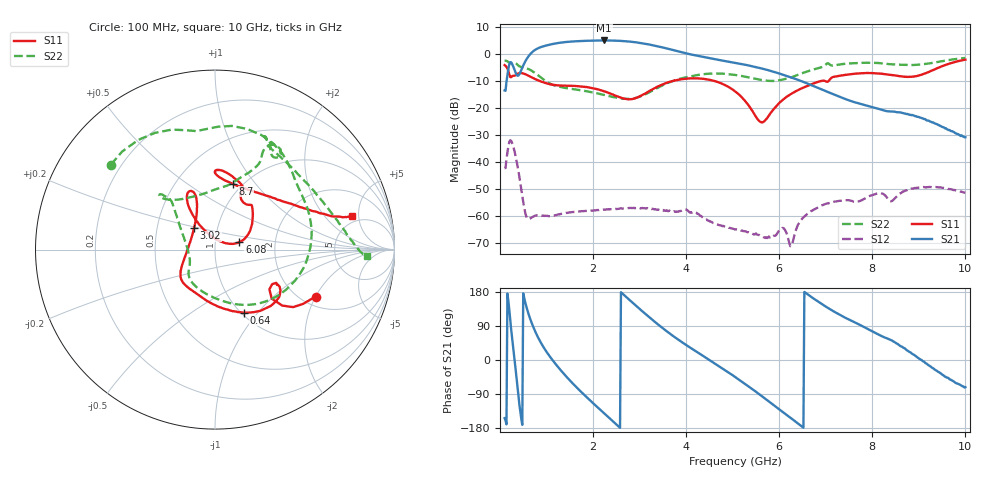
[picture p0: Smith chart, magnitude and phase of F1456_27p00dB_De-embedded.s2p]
! Integrated Device Technology
! Corporate Headquarters
! 6024 Silver Creek Valley Road
! San Jose, CA 95138  USA
! Phone:  1-408-284-8200
! Toll Free:  1-800-223-1366
! Webpage:  http://www.idt.com/
! Timing and RF Division
! 515 Groton Road, Suite 102
! Westford, MA 01886-6024
! Device:  F1456
! Description: 6-bit 0.5 dB Transmit Variable Gain Amplifier
! Frequency:  2100.0 -  2950.00 MHz
! Package:  6x6 mm Thin QFN Plastic Package: 28 pin
! State:  54
! Atten State:  27.0 dB
! Voltage:  +5.00 Volts
! Current:  216.965 mA
! Data:  The device was measured on a the F1455 evaluation board which has
!  individual transmission lines to the RF pins.  Data was collected
!  using a calibrated network analyzer.  The evaluation board was
!  de-embedded using a TRL calibration technique.
!  The reference plane is the edge of the package pin.
!  Pin  1 = CSb
!  Pin  2 = DATA
!  Pin  3 = CLK
!  Pin  4 = RSET
!  Pin  5 = GND
!  Pin  6 = RFIN  = Port 1
!  Pin  7 = GND
!  Pin  8 = NC
!  Pin  9 = NC
!  Pin 10 = NC
!  Pin 11 = NC
!  Pin 12 = NC
!  Pin 13 = NC
!  Pin 14 = /STBY
!  Pin 15 = GND
!  Pin 16 = RFOUT  = Port 2
!  Pin 17 = GND
!  Pin 18 = NC
!  Pin 19 = NC
!  Pin 20 = NC
!  Pin 21 = GND
!  Pin 22 = NC
!  Pin 23 = GND
!  Pin 24 = NC
!  Pin 25 = NC
!  Pin 26 = NC
!  Pin 27 = GND
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# GHz S dB R 50
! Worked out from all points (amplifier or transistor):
!   496 points, 100 MHz to 10 GHz, reference 50 ohm
!   highest |S21| = 5.0 dB at 2.24 GHz (marker M1)
!   |S21| within 3 dB of that: 805.4 MHz to 3.593 GHz (2.787 GHz wide, 127 % of centre)
!   unconditionally stable (mu >= 1): start of sweep to end of sweep
!   at 1.74 GHz: K = 210.59, MAG = 5.3 dB, |S12| = -58.3 dB
!   at 5.06 GHz: K = 1041.17, MAG = -2.3 dB, |S12| = -65.1 dB
!   at 10 GHz: K = 708.50, MAG = -21.2 dB, |S12| = -51.4 dB
!   S11 on the Smith chart (normalised r, x): 100 MHz: 2.37, -2.03; 640 MHz: 1.03, -0.85; 3.02 GHz: 0.77, +0.19; 6.08 GHz: 1.31, +0.11; 8.7 GHz: 0.90, +0.78; 10 GHz: 4.19, +4.12
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0.1  -4.12 -24.9  -13.50 -153.5  -42.30 50.1  -2.51 140.8
0.24  -8.59 -31.1  -3.07 82.0  -32.17 -77.3  -3.45 94.6
0.32  -7.99 -29.1  -6.16 -5.9  -36.59 -155.6  -3.24 67.9
0.42  -7.04 -36.6  -7.42 -120.2  -45.85 139.0  -4.59 40.6
0.52  -7.35 -50.8  -3.54 164.1  -56.88 119.2  -5.04 19.9
0.64  -8.27 -65.5  -0.25 111.9  -61.05 142.8  -5.80 -7.6
0.82  -9.76 -83.9  2.15 59.2  -59.76 119.8  -7.88 -45.7
1.14  -11.44 -110.6  3.74 -1.9  -59.92 83.2  -11.45 -91.3
1.76  -12.03 -139.0  4.84 -86.0  -58.21 48.3  -13.49 -132.6
2.24  -13.83 -154.4  5.03 -141.0  -57.69 30.3  -15.17 -145.4
2.62  -16.33 -179.9  4.84 176.7  -57.22 16.4  -16.52 -160.5
3.02  -15.55 134.5  4.09 132.7  -57.21 -1.5  -15.66 169.3
3.4  -11.98 113.6  2.82 93.4  -57.60 -17.8  -12.45 145.4
4.1  -9.02 112.7  -0.16 31.7  -58.61 -50.9  -8.26 132.3
5.06  -13.92 123.0  -3.27 -45.4  -65.05 -102.0  -7.76 135.5
5.62  -25.31 66.2  -5.35 -94.8  -67.47 -165.5  -9.62 120.3
6.08  -16.94 17.0  -7.69 -137.7  -64.50 154.2  -9.44 88.6
6.26  -14.74 21.4  -8.72 -154.1  -70.99 160.9  -8.64 77.8
6.7  -11.15 40.7  -11.60 165.5  -58.09 146.0  -5.92 64.1
8.36  -7.62 88.6  -21.26 54.9  -54.25 60.1  -3.75 62.5
8.7  -8.40 75.0  -22.07 30.4  -50.62 67.3  -4.04 51.3
10  -2.09 13.8  -30.84 -71.8  -51.42 -26.9  -1.46 -2.6
